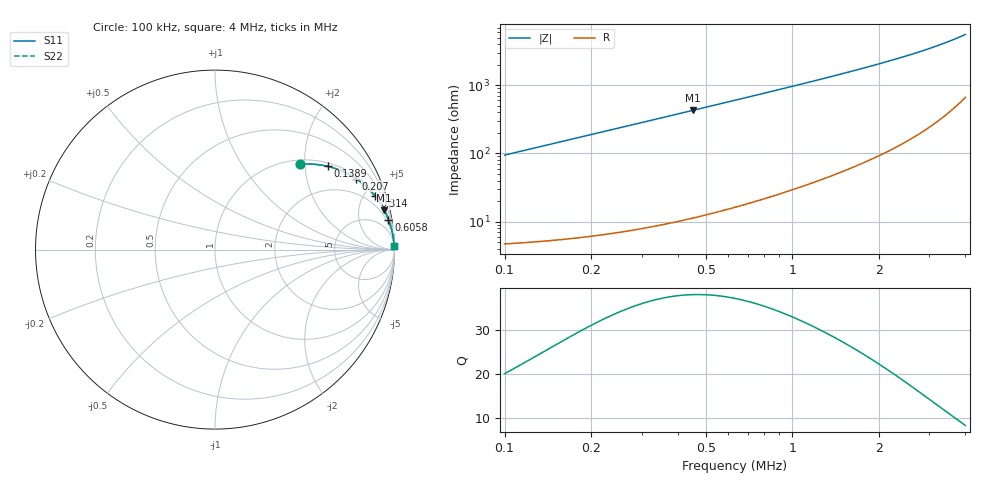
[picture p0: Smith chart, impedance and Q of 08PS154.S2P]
! Coilcraft 0805PS-154 Power Chip Inductor
! 5 February 2003
# MHZ S MA R 50
!Freq  MagS11  AngS11  MagS21  AngS21  MagS12  AngS12  MagS22  AngS22
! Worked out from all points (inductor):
!   402 points, 100 kHz to 4 MHz, reference 50 ohm
!   read as one part in series: L = 150 uH near 119.5 kHz
!   highest Q = 38 at 450.1 kHz (marker M1), where L = 151 uH
!   S11 on the Smith chart (normalised r, x): 100 kHz: 1.09, +1.89; 138.9 kHz: 1.10, +2.62; 207 kHz: 1.12, +3.90; 314 kHz: 1.16, +5.93; 605.8 kHz: 1, +12; 4 MHz: open
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0.1  0.6699 45.1  0.7098 -42.0  0.7098 -42.0  0.6699 45.1
0.119452  0.7323 40.5  0.6497 -47.0  0.6497 -47.0  0.7323 40.5
0.138904  0.7803 36.5  0.5954 -51.2  0.5954 -51.2  0.7803 36.5
0.168082  0.8327 31.7  0.5251 -56.3  0.5251 -56.3  0.8327 31.7
0.187534  0.8585 29.0  0.4851 -59.1  0.4851 -59.1  0.8585 29.0
0.206986  0.8789 26.7  0.45 -61.5  0.45 -61.5  0.8789 26.7
0.255616  0.9144 22.3  0.379 -66.1  0.379 -66.1  0.9144 22.3
0.313972  0.9398 18.5  0.3169 -70.0  0.3169 -70.0  0.9398 18.5
0.372328  0.9552 15.7  0.2714 -72.7  0.2714 -72.7  0.9552 15.7
0.450136  0.9679 13.1  0.2272 -75.4  0.2272 -75.4  0.9679 13.1
0.527944  0.9757 11.2  0.195 -77.2  0.195 -77.2  0.9757 11.2
0.605752  0.9808 9.8  0.1705 -78.7  0.1705 -78.7  0.9808 9.8
0.751642  0.9866 7.9  0.1377 -80.5  0.1377 -80.5  0.9867 7.9
0.887806  0.9898 6.7  0.1164 -81.6  0.1164 -81.6  0.9898 6.7
1.043422  0.9921 5.7  0.09866 -82.6  0.09866 -82.6  0.9921 5.7
1.21849  0.9937 4.8  0.08393 -83.3  0.08393 -83.3  0.9937 4.8
1.403284  0.9948 4.1  0.07222 -83.8  0.07222 -83.8  0.9948 4.1
1.70479  0.996 3.3  0.05834 -84.4  0.05834 -84.4  0.996 3.3
2.054926  0.9967 2.7  0.04706 -84.7  0.04706 -84.7  0.9967 2.7
2.706568  0.9974 1.9  0.03331 -84.6  0.03331 -84.6  0.9974 1.9
3.35821  0.9977 1.4  0.02436 -83.8  0.02436 -83.8  0.9977 1.4
4  0.9977 1.0  0.01799 -82.1  0.01799 -82.1  0.9977 1.0
